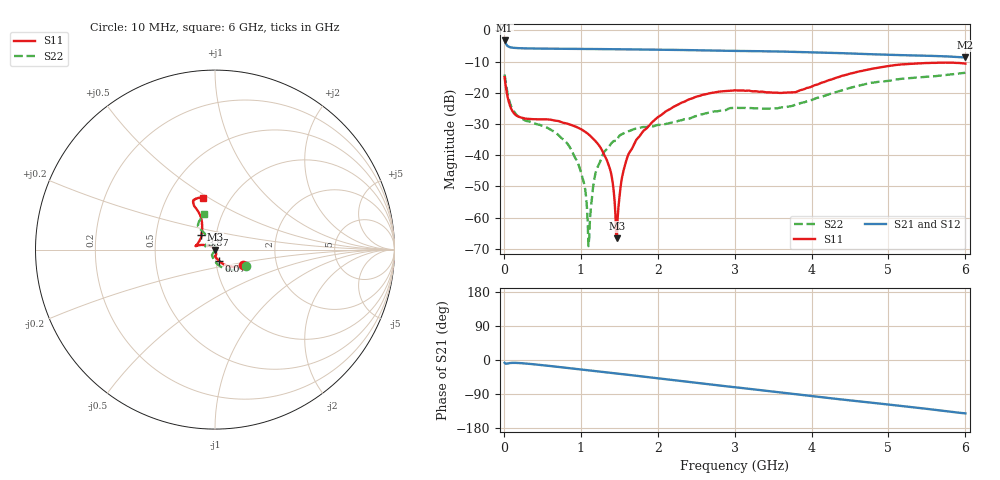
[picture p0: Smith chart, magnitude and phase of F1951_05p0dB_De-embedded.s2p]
! Integrated Device Technology
! Corporate Headquarters
! 6024 Silver Creek Valley Road
! San Jose, CA 95138  USA
! Phone:  1-408-284-8200
! Toll Free:  1-800-223-1366
! Webpage:  http://www.idt.com/
! Timing and RF Division
! 515 Groton Road, Suite 102
! Westford, MA 01886-6024
! Device:  F1951
! Description: 6-bit 0.5 dB Digital Step Attenuator
! Frequency:  100.0 -  4000.00 MHz
! Package:  4x4 mm Thin QFN Plastic Package: 24 pin
! Ports:  2 RF, 6 DC
!  Pin  1  = NC
!  Pin  2  = RF1  =  Port 1
!  Pin  3  = GND
!  Pin  4  = NC
!  Pin  5  = Serial Data Out (SDO)
!  Pin  6  = NC
!  Pin  7  = Reset Bar ( RSTb)
!  Pin  8  = Clock (CLK)
!  Pin  9  = Chip Select Bar (CSb)
!  Pin 10  = NC
!  Pin 11  = Serial Data In (SDI)
!  Pin 12  = NC
!  Pin 13  = NC
!  Pin 14  = VDD
!  Pin 15  = NC
!  Pin 16  = GND
!  Pin 17  = RF2  =  Port 2
!  Pin 18  = NC
!  Pin 19  = GND
!  Pin 20  = GND
!  Pin 21  = GND
!  Pin 22  = GND
!  Pin 23  = GND
!  Pin 24  = GND
! State:  10
! Atten State:  5.0 dB
! Voltage:  +3.30 Volts
! Current:  0.474 mA
! Data:  The device was measured on a F195X evaluation board which has
!  individual transmission lines to the RF pins.  Data was collected
!  de-embedded using a Automatic Fixture Removal [AFR] (Keysight Technologies).
!  The reference plane is the edge of the package pin.
! Misc:  Lot Code  1225BCA
!  Action Tracker AT0399
! Date Measured:  2018-09-13
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# GHz S dB R 50
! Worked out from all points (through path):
!   600 points, 10 MHz to 6 GHz, reference 50 ohm
!   highest |S21| = -3.24 dB at 10 MHz (marker M1); lowest = -8.7 dB at 6 GHz (marker M2)
!   group delay of S21, straight-line fit = 64 ps
!   lowest |S11| = -66.6 dB at 1.47 GHz (marker M3), VSWR 1.00, Z = 50 + j0.0338 ohm
!   |S11| at or under -10 dB: start of sweep to end of sweep
!   |S22| runs from -69.2 to -13.6 dB; largest |S21 - S12| = 0.0007
!   S11 on the Smith chart (normalised r, x): 10 MHz: 1.34, -0.25; 70 MHz: 1.04, -0.13; 3.87 GHz: 0.85, +0.14; 6 GHz: 0.75, +0.47
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0.01  -14.99 -29.8  -3.24 -7.5  -3.24 -7.5  -14.14 -28.3
0.07  -23.37 -69.8  -5.32 -8.3  -5.32 -8.4  -22.54 -84.2
0.21  -27.83 -87.4  -5.73 -8.2  -5.73 -8.2  -27.92 -112.4
0.8  -29.74 -83.1  -5.92 -20.3  -5.92 -20.3  -35.56 -117.8
1.01  -31.75 -73.9  -5.97 -25.1  -5.98 -25.1  -46.20 -108.6
1.05  -32.37 -73.4  -5.98 -26.0  -5.98 -25.9  -49.87 -106.2
1.09  -33.09 -72.0  -5.99 -26.9  -5.99 -26.8  -61.59 -78.4
1.11  -33.51 -71.1  -5.99 -27.3  -5.99 -27.3  -66.32 52.3
1.17  -34.95 -69.0  -6.00 -28.7  -6.00 -28.7  -48.69 69.0
1.21  -36.02 -68.0  -6.00 -29.6  -6.00 -29.6  -44.39 76.7
1.38  -44.46 -53.1  -6.03 -33.6  -6.03 -33.6  -36.78 78.0
1.45  -58.91 -48.4  -6.06 -35.3  -6.06 -35.3  -35.43 79.9
1.47  -66.63 46.5  -6.07 -35.7  -6.07 -35.7  -35.29 84.0
1.54  -46.69 119.5  -6.07 -37.2  -6.07 -37.2  -33.21 85.2
1.62  -39.72 127.0  -6.09 -39.2  -6.09 -39.2  -32.33 86.5
2.01  -27.67 148.4  -6.20 -48.5  -6.20 -48.5  -30.29 110.5
2.49  -21.35 162.7  -6.37 -59.9  -6.37 -59.9  -27.53 147.4
3.01  -19.22 169.6  -6.58 -72.0  -6.59 -71.9  -24.81 158.6
3.87  -19.08 133.4  -6.94 -92.0  -6.94 -92.0  -23.24 125.2
4.01  -17.90 124.3  -7.02 -95.4  -7.02 -95.4  -22.26 122.4
5.01  -11.42 115.5  -7.85 -117.7  -7.85 -117.7  -16.18 126.0
6  -10.65 102.9  -8.69 -140.8  -8.69 -140.8  -13.59 106.9
